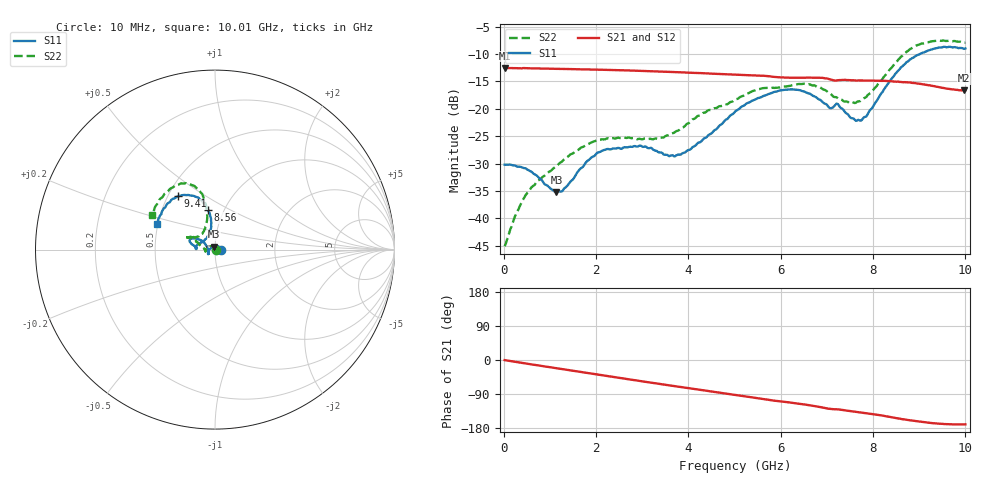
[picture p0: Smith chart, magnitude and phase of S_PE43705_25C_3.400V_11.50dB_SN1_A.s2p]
! Device ID: PE43705
! Serial: 1
! Insertion: A
! Impedance: 50 ohm
! Temp: 25C
! VDD: 3.400V
! Attenuation Step: 11.50dB
#  Hz  S  RI  R  50
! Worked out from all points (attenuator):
!   401 points, 10 MHz to 10.01 GHz, reference 50 ohm
!   highest |S21| = -12.52 dB at 10 MHz (marker M1); lowest = -16.6 dB at 9.985 GHz (marker M2)
!   lowest |S11| = -35.2 dB at 1.135 GHz (marker M3), VSWR 1.04, Z = 49.5 + j1.66 ohm
!   |S11| at or under -10 dB: start of sweep to 9.021 GHz
!   |S22| runs from -45.1 to -7.5 dB; largest |S21 - S12| = 0.0022
!   S11 on the Smith chart (normalised r, x): 10 MHz: 1.06, +0.00; 8.56 GHz: 0.84, +0.39; 9.41 GHz: 0.56, +0.39; 10.01 GHz: 0.49, +0.16
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1e7  0.0309 0.000215  0.2367 -0.00106  0.2368 -0.000987  0.00557 0.000381
4.6e8  0.0245 0.015  0.2321 -0.0369  0.2322 -0.0364  0.00143 0.0161
1.135e9  -0.0047 0.0168  0.2154 -0.0858  0.2155 -0.0857  -0.0233 0.0187
1.31e9  -0.0133 0.0135  0.2098 -0.0978  0.2098 -0.0976  -0.0309 0.0162
1.685e9  -0.029 0.00194  0.1948 -0.1217  0.1948 -0.1215  -0.0441 0.00714
2.21e9  -0.0396 -0.0159  0.1694 -0.1511  0.1695 -0.151  -0.053 -0.00604
2.96e9  -0.0388 -0.0251  0.1254 -0.1836  0.1256 -0.1834  -0.0527 -0.00691
3.36e9  -0.035 -0.0197  0.0999 -0.1953  0.1002 -0.195  -0.0535 -0.0036
3.885e9  -0.0396 0.00138  0.0652 -0.205  0.0654 -0.2049  -0.0669 0.0108
5.01e9  -0.0785 0.0524  -0.00788 -0.2048  -0.00773 -0.205  -0.1109 0.0494
5.51e9  -0.1096 0.0616  -0.0387 -0.1978  -0.0386 -0.1979  -0.1358 0.0657
5.985e9  -0.1344 0.0605  -0.0632 -0.1834  -0.0623 -0.1836  -0.1411 0.0684
6.685e9  -0.1296 0.0305  -0.098 -0.1657  -0.0982 -0.1657  -0.149 0.0683
7.41e9  -0.0856 0.0341  -0.1254 -0.1345  -0.1246 -0.1348  -0.0866 0.0781
7.71e9  -0.052 0.0592  -0.1351 -0.1217  -0.1346 -0.1216  -0.0652 0.0976
7.885e9  -0.0339 0.082  -0.1406 -0.1144  -0.1405 -0.115  -0.0543 0.1213
8.36e9  -0.023 0.1759  -0.1552 -0.0898  -0.1546 -0.0902  -0.0463 0.2216
8.56e9  -0.0378 0.2221  -0.16 -0.0764  -0.1586 -0.0774  -0.0571 0.2776
8.935e9  -0.0931 0.2903  -0.1624 -0.0553  -0.1618 -0.0543  -0.1202 0.3572
9.41e9  -0.2046 0.2976  -0.1553 -0.0335  -0.155 -0.0335  -0.2199 0.359
9.985e9  -0.3186 0.1515  -0.145 -0.0257  -0.145 -0.0262  -0.3446 0.2059
1.001e10  -0.3257 0.143  -0.1454 -0.0262  -0.1459 -0.027  -0.3523 0.1948
